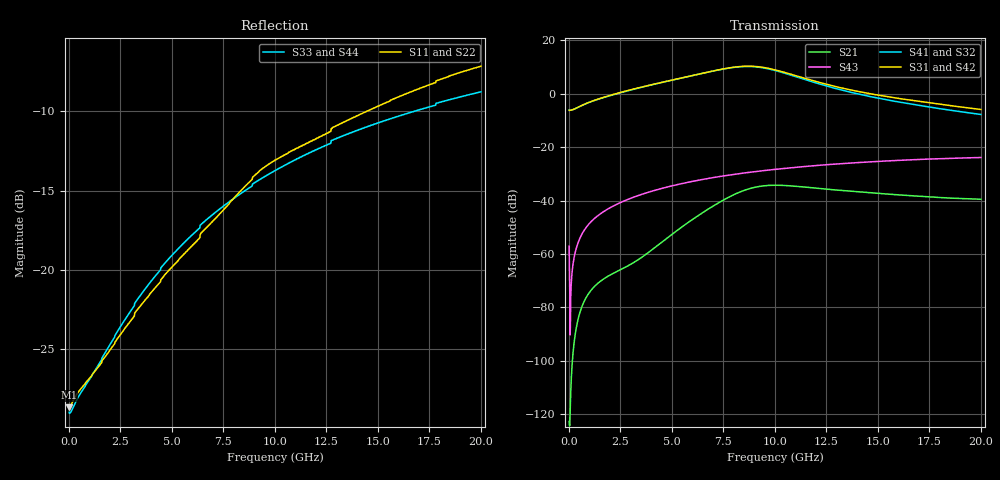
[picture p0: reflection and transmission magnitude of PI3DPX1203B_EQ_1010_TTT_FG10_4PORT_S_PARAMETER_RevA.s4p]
! NPort=4 DATA=2000 NOISE=0 GROUPDELAY=0 COMPLEX_DATAFORMAT=POLAR
! NumOfBlock=1 NumOfParam=0
! .MODEL Smodel S TSTONEFILE=PI3DPX1203B_EQ_1010_TTT_FG10_4PORT_S_PARAMETER_RevA.s4p TYPE=S
!  -- The above .MODEL line can be used for the S element in the netlist.
! The s parameter is extracted from the linear redriver, it is not bi-directional; only s(4,1)s(4,2) and s(3,1)s(3,2)
! should be the insertion loss
!Port definition:
!Port1 = input+
!Port2 = input-
!Port3 = output+
!Port4 = output-
# Hz S MA R  50
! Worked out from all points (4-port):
!   2000 points, 10 MHz to 20 GHz, reference 50 ohm
!   strongest paths, dB at 10 MHz, 5.01 GHz, 10.01 GHz, 15.01 GHz, 20 GHz:
!     S31: -6.2, 5.2, 9.0, -0.5, -5.9
!     S42: -6.2, 5.2, 9.0, -0.5, -5.8
!     S41: -6.2, 5.1, 8.8, -1.6, -7.7
!     S32: -6.2, 5.1, 8.7, -1.6, -7.7
!     S43: -57.1, -34.4, -28.3, -25.3, -23.8
!     S21: -122.7, -52.6, -34.2, -37.3, -39.5
!   lowest |S11| = -28.6 dB at 10 MHz (marker M1), VSWR 1.08, Z = 46.4 - j0.0306 ohm
!   |S11| at or under -10 dB: start of sweep to 14.46 GHz
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1e7  0.03701 -179.5  7.338e-07 10.6  0 0.0  0 0.0
     7.338e-07 10.6  0.03701 -179.5  0 0.0  0 0.0
     0.4917 -0.0  0.4917 180.0  0.03566 178.2  0.001403 -77.8
     0.4917 180.0  0.4917 -0.0  0.001403 -77.8  0.03566 178.2
3.09e9  0.0705 -126.8  0.0006748 136.5  1.535e-10 56.1  2.638e-09 107.3
        0.0006743 136.5  0.0705 -126.8  2.638e-09 107.3  1.535e-10 56.0
        1.217 0.6  1.204 -178.2  0.07578 -126.6  0.01143 77.7
        1.204 -178.2  1.217 0.6  0.01143 77.7  0.07578 -126.6
5.88e9  0.1174 -110.9  0.004135 152.4  1.324e-08 -121.0  1.192e-07 68.6
        0.004134 152.5  0.1174 -110.9  1.192e-07 68.6  1.325e-08 -121.0
        2.154 -40.6  2.152 140.9  0.127 -117.2  0.02249 65.7
        2.153 140.9  2.154 -40.6  0.02249 65.7  0.127 -117.2
8.26e9  0.1752 -105.1  0.01431 110.6  3.225e-07 156.0  8.971e-07 19.4
        0.01431 110.7  0.1752 -105.1  8.963e-07 19.4  3.228e-07 156.1
        3.235 -99.0  3.205 82.3  0.1726 -115.9  0.03203 53.6
        3.206 82.3  3.235 -99.0  0.03203 53.6  0.1726 -115.9
9.79e9  0.2172 -107.2  0.01938 67.0  1.099e-06 94.8  1.862e-06 -18.2
        0.01937 67.0  0.2171 -107.2  1.86e-06 -18.2  1.099e-06 94.8
        2.946 -148.9  2.873 32.2  0.2018 -116.2  0.03773 45.5
        2.875 32.2  2.945 -148.9  0.03773 45.5  0.2018 -116.2
1.201e10  0.2592 -109.2  0.01718 25.6  2.899e-06 29.5  3.608e-06 -46.4
          0.01714 25.8  0.2592 -109.2  3.609e-06 -46.3  2.901e-06 29.5
          1.697 163.1  1.593 -15.5  0.2393 -117.5  0.04549 34.1
          1.595 -15.5  1.696 163.1  0.04549 34.1  0.2393 -117.5
2e10  0.4382 -117.5  0.01057 -17.6  2.235e-05 -108.9  3.147e-05 -133.8
      0.01063 -17.2  0.4383 -117.5  3.154e-05 -133.8  2.238e-05 -108.8
      0.5096 75.7  0.411 -91.2  0.3637 -123.9  0.06431 -7.1
      0.4109 -91.4  0.5104 75.8  0.06431 -7.1  0.3637 -123.9
